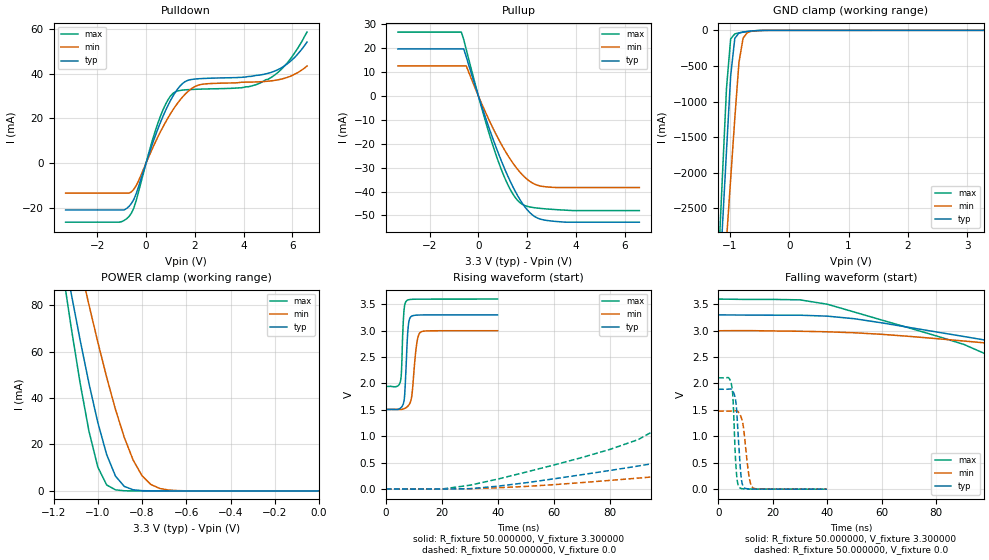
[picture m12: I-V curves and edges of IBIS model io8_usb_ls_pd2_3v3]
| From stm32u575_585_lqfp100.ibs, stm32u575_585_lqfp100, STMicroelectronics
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|   Model io8_usb_ls_pd2_3v3
[Model]  io8_usb_ls_pd2_3v3
Model_type I/O
Polarity   Non-Inverting
Enable   Active-Low
Vinl =   0.990000V
Vinh =   2.310000V
Vmeas =  1.650000V
Cref =   50.000000pF
Rref =   100.000000M
Vref =   0.0V
C_comp   7.156600pF   7.055100pF   7.302500pF
[Temperature Range]   25.000000   0.140000k   -40.000000
[Pullup Reference]   3.300000V   3.000000V   3.600000V
[Pulldown Reference]   0.0V   0.0V   0.0V
[POWER Clamp Reference]   3.300000V   3.000000V   3.600000V
[GND Clamp Reference]   0.0V   0.0V   0.0V
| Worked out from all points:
|   slope of the pulldown table from 0 to 0.495 V, typ, clamps not added: 31.7 ohm
|   slope of the pullup table from 0 to 0.495 V, typ, clamps not added: 32.9 ohm
|   GND clamp passes 1 mA (typ) near -0.45 V on its own axis
|   POWER clamp passes 1 mA (typ) near -0.85 V on its own axis
|   rising waveform, R_fixture 50.000000, V_fixture 3.300000: 20-80 % time 968ps typ, 1.53ns min, 711ps max; typ from 1.51 V to 3.3 V
|   rising waveform, R_fixture 50.000000, V_fixture 0.0: 20-80 % time 81.8ns typ, 127ns min, 54.5ns max; typ from 0 V to 1.89 V
|   falling waveform, R_fixture 50.000000, V_fixture 3.300000: 20-80 % time 79.4ns typ, 125ns min, 50.9ns max; typ from 3.3 V to 1.51 V
|   falling waveform, R_fixture 50.000000, V_fixture 0.0: 20-80 % time 1.41ns typ, 1.93ns min, 1.08ns max; typ from 1.89 V to 0 V
[Pulldown]
|Voltage   I(typ)   I(min)   I(max)
-3.3V     -21.02mA   -13.49mA   -26.5mA
-1.1V     -21.02mA   -13.49mA   -26.5mA
-700mV    -19.42mA   -13.49mA   -23.95mA
-500mV    -16.23mA   -11.71mA   -20.06mA
300mV     9.809mA    7.466mA    11.69mA
700mV     21.12mA    16.34mA    23.99mA
1.1V      29.97mA    23.81mA    31.21mA
1.6V      36.5mA     30.84mA    32.8mA
2.3V      37.88mA    35.3mA     33.16mA
5V        40.21mA    36.69mA    37.55mA
5.8V      44.54mA    38.44mA    45.04mA
6.6V      54.2mA     43.5mA     58.7mA
[Pullup]
|Voltage   I(typ)   I(min)   I(max)
-3.3V     19.6mA     12.52mA    26.65mA
-700mV    19.6mA     12.52mA    26.65mA
-600mV    19.6mA     12.52mA    23.46mA
-500mV    16.36mA    12.52mA    19.44mA
200mV     -6.335mA   -4.782mA   -7.46mA
700mV     -20.86mA   -15.62mA   -24.03mA
1.2V      -33.4mA    -24.78mA   -37.01mA
1.5V      -39.72mA   -29.3mA    -42.37mA
1.7V      -43.31mA   -31.86mA   -44.63mA
2.2V      -49.66mA   -36.35mA   -46.62mA
2.7V      -51.91mA   -37.96mA   -47.2mA
6.6V      -52.82mA   -38.34mA   -47.98mA
[GND_clamp]
|Voltage   I(typ)   I(min)   I(max)
-3.3V     -9.287A    -9.833A    -9.745A
-1.2V     -3.857A    -4.664A    -3.345A
-1.13V    -2.774A    -3.805A    -2.072A
-1.06V    -1.695A    -2.947A    -813.1mA
-990mV    -641.8mA   -2.091A    -120.9mA
-920mV    -113.3mA   -1.238A    -49.91mA
-850mV    -36.82mA   -452mA     -36.33mA
-780mV    -22.67mA   -108.9mA   -26.24mA
-710mV    -15.24mA   -32.28mA   -17.46mA
-570mV    -5.138mA   -7.046mA   -4.93mA
-360mV    -107.9uA   -475uA     -47.23uA
3.28V     163.3uA    123.6uA    195.4uA
[POWER_clamp]
|Voltage   I(typ)   I(min)   I(max)
-3.28V    1.355A     1.167A     1.664A
-1.16V    105.7mA    131.6mA    95.69mA
-1.12V    84.97mA    114mA      70.27mA
-1.08V    65.05mA    96.83mA    46.54mA
-1.04V    46.34mA    80.15mA    25.76mA
-1V       29.51mA    64.13mA    10.3mA
-960mV    15.69mA    48.99mA    2.571mA
-920mV    6.373mA    35.1mA     455.6uA
-840mV    490.7uA    13.24mA    11.36uA
-760mV    27.33uA    2.767mA    754.7nA
-640mV    348.1nA    134.1uA    754.7nA
0V        0A         50.53nA    0A
[Ramp]
| variable   typ   min   max
dV/dt_r  1.13454/81.36436n   0.88644/0.12622u   1.26420/54.15103n
dV/dt_f  1.07436/79.05580n   0.89364/0.12510u   0.99276/50.90040n
R_load = 50.000000
[Rising Waveform]
R_fixture= 50.000000
V_fixture= 3.300000
V_fixture_min= 3.000000
V_fixture_max= 3.600000
|time   V(typ)   V(min)   V(max)
0s        1.508V     1.509V     1.943V
5.205ns   1.532V     1.507V     2.038V
5.606ns   1.552V     1.508V     2.265V
6.326ns   1.632V     1.518V     3.27V
6.807ns   1.861V     1.529V     3.502V
7.928ns   3.042V     1.573V     3.581V
8.969ns   3.265V     1.682V     3.592V
10.89ns   3.293V     2.703V     3.595V
12.25ns   3.296V     2.966V     3.596V
39.88ns   3.298V     2.998V     3.598V
[Rising Waveform]
R_fixture= 50.000000
V_fixture= 0.0
V_fixture_min= 0.0
V_fixture_max= 0.0
|time   V(typ)   V(min)   V(max)
0s        53.49nV    540.6nV    167.3nV
30.03ns   4.926mV    5.759mV    71.79mV
70.07ns   271.6mV    121.5mV    597mV
90.09ns   435.4mV    206.1mV    936mV
110.1ns   617.5mV    299.2mV    1.628V
130.1ns   837.3mV    398.5mV    2.058V
170.2ns   1.603V     617.4mV    2.214V
260.3ns   1.913V     1.324V     2.213V
380.4ns   1.913V     1.458V     2.2V
4.985us   1.891V     1.478V     2.107V
[Falling Waveform]
R_fixture= 50.000000
V_fixture= 3.300000
V_fixture_min= 3.000000
V_fixture_max= 3.600000
|time   V(typ)   V(min)   V(max)
0s        3.298V     2.998V     3.598V
40.04ns   3.274V     2.978V     3.499V
90.09ns   2.889V     2.804V     2.739V
120.1ns   2.613V     2.662V     1.905V
140.1ns   2.361V     2.562V     1.766V
170.2ns   1.738V     2.394V     1.778V
200.2ns   1.533V     2.161V     1.802V
270.3ns   1.49V      1.654V     1.844V
400.4ns   1.496V     1.519V     1.891V
4.985us   1.508V     1.509V     1.943V
[Falling Waveform]
R_fixture= 50.000000
V_fixture= 0.0
V_fixture_min= 0.0
V_fixture_max= 0.0
|time   V(typ)   V(min)   V(max)
0s        1.891V     1.478V     2.107V
4.885ns   1.89V      1.479V     1.974V
5.445ns   1.85V      1.482V     1.7V
6.647ns   1.57V      1.484V     341.9mV
7.768ns   671.8mV    1.431V     34.1mV
8.408ns   231.7mV    1.363V     13.73mV
9.049ns   64.09mV    1.238V     7.337mV
11.21ns   4.811mV    276.1mV    2.724mV
12.57ns   2.639mV    32.94mV    1.908mV
39.88ns   53.49nV    540.6nV    167.3nV
